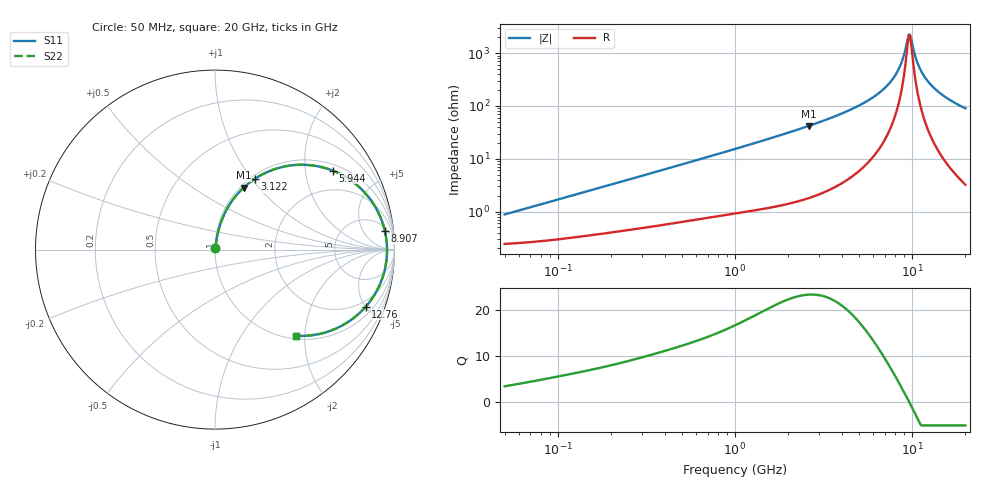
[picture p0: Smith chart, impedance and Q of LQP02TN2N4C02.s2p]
!Murata Part Number: LQP02TN2N4C02
!These Parameters are Measured in Series Mode Connection
!  o--[Z]--o
!Port1  Port2
!  o-------o
!Freq. Start=50[MHz] Stop=20[GHz], 401[Steps]
# Hz S RI R 50
!Freq.(Hz) S11(Real) S11(Imag) S21(Real) S21(Imag) S12(Real) S12(Imag) S22(Real) S22(Imag)
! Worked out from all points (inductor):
!   401 points, 50 MHz to 20 GHz, reference 50 ohm
!   read as one part in series: L = 2.68 nH near 51.52 MHz
!   highest Q = 23.3 at 2.608 GHz (marker M1), where L = 2.55 nH
!   self-resonance near 9.6 GHz
!   S11 on the Smith chart (normalised r, x): 50 MHz: 1.00, +0.02; 3.122 GHz: 1.04, +1.04; 5.944 GHz: 1.21, +2.83; 8.907 GHz: 7, +15; 12.76 GHz: 1.53, -5.02; 20 GHz: 1.06, -1.80
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5e7  0.0025 0.00842  0.9975 -0.00842  0.9975 -0.00842  0.0025 0.00842
1.364002e8  0.00385 0.0222  0.9961 -0.0222  0.9961 -0.0222  0.00385 0.0222
3.721004e8  0.00873 0.0576  0.9913 -0.0576  0.9913 -0.0576  0.00873 0.0576
1e9  0.0313 0.1468  0.9687 -0.1468  0.9687 -0.1468  0.0313 0.1468
1.740566e9  0.0775 0.245  0.9225 -0.245  0.9225 -0.245  0.0775 0.245
2.608132e9  0.1597 0.3456  0.8403 -0.3456  0.8403 -0.3456  0.1597 0.3456
2.728004e9  0.1734 0.3578  0.8266 -0.3578  0.8266 -0.3578  0.1734 0.3578
3.121702e9  0.2217 0.3943  0.7783 -0.3943  0.7783 -0.3943  0.2217 0.3943
4.608136e9  0.4425 0.471  0.5575 -0.471  0.5575 -0.471  0.4425 0.471
5.944466e9  0.6571 0.4397  0.3429 -0.4397  0.3429 -0.4397  0.6571 0.4397
7.442007e9  0.8505 0.2987  0.1495 -0.2987  0.1495 -0.2987  0.8505 0.2987
8.264682e9  0.9169 0.1914  0.0831 -0.1914  0.0831 -0.1914  0.9169 0.1914
8.907419e9  0.9466 0.1023  0.0534 -0.1023  0.0534 -0.1023  0.9466 0.1023
9.457416e9  0.9575 0.0268  0.0425 -0.0268  0.0425 -0.0268  0.9575 0.0268
9.745021e9  0.9584 -0.0116  0.0416 0.0116  0.0416 0.0116  0.9584 -0.0116
9.892087e9  0.9577 -0.0308  0.0423 0.0308  0.0423 0.0308  0.9577 -0.0308
1.050288e10  0.9472 -0.1065  0.0528 0.1065  0.0528 0.1065  0.9472 -0.1065
1.098561e10  0.9316 -0.1612  0.0684 0.1612  0.0684 0.1612  0.9316 -0.1612
1.166392e10  0.9016 -0.2293  0.0984 0.2293  0.0984 0.2293  0.9016 -0.2293
1.276073e10  0.8402 -0.3178  0.1598 0.3178  0.1598 0.3178  0.8402 -0.3178
1.550395e10  0.6702 -0.4416  0.3298 0.4416  0.3298 0.4416  0.6702 -0.4416
2e10  0.4503 -0.48  0.5497 0.48  0.5497 0.48  0.4503 -0.48
